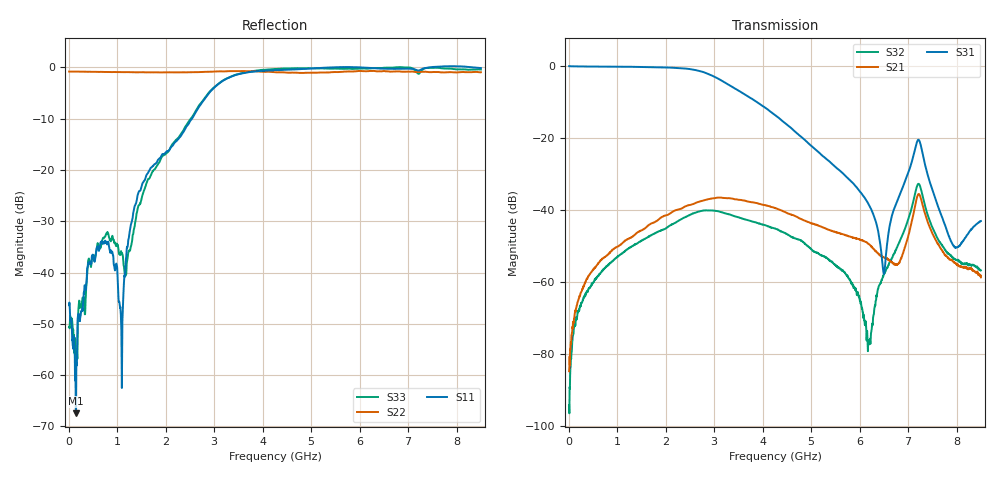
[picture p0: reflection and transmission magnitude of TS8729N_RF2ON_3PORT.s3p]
!Created with skrf (http://scikit-rf.org).
# GHz S RI R 50.0
!freq ReS11 ImS11 ReS12 ImS12 ReS13 ImS13
! ReS21 ImS21 ReS22 ImS22 ReS23 ImS23
! ReS31 ImS31 ReS32 ImS32 ReS33 ImS33
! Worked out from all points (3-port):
!   1601 points, 10 MHz to 8.5 GHz, reference 50 ohm
!   strongest paths, dB at 10 MHz, 2.132 GHz, 4.255 GHz, 6.378 GHz, 8.5 GHz:
!     S31: -0.1, -0.5, -13.6, -45.5, -43.0
!     S21: -84.7, -40.6, -39.4, -52.0, -58.6
!     S32: -94.2, -43.9, -45.1, -61.8, -56.7
!   lowest |S11| = -67.4 dB at 153.3 MHz (marker M1), VSWR 1.00, Z = 50 + j0.0217 ohm
!   |S11| at or under -10 dB: start of sweep to 2.545 GHz
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0.01  0.00455 0.00155  -1.17e-05 4.26e-05  0.9927 -0.0113
      1.37e-05 5.65e-05  -0.9094 0.00493  1.37e-05 -2.45e-05
      0.9926 -0.0114  1.9e-05 4.24e-06  0.0022 0.00197
0.1532688  -0.000365 0.000217  3.07e-05 0.000416  0.9783 -0.1229
           3.89e-05 0.000436  -0.9076 0.0485  -4.84e-05 -0.000292
           0.9783 -0.1229  -4.95e-05 -0.00031  0.000347 -0.00126
1.697388  -0.1028 -0.022  0.000863 0.00644  0.149 -0.9512
          0.000857 0.00644  -0.776 0.4434  -0.00366 0.00252
          0.1489 -0.951  -0.00367 0.00255  -0.0887 -0.006
2.742719  -0.1807 0.411  0.00942 0.00952  -0.7252 -0.4158
          0.00942 0.00949  -0.5471 0.7168  0.00281 0.00936
          -0.7254 -0.4141  0.00279 0.00935  -0.2199 0.401
4.255  0.8445 0.4066  0.00998 -0.00391  -0.1088 0.1781
       0.00998 -0.00389  -0.2796 0.8523  0.00531 -0.00151
       -0.1088 0.1775  0.00536 -0.00151  0.8125 0.5204
6.186475  0.9781 -0.1507  0.0026 -0.00221  -0.000502 0.012
          0.00258 -0.00221  0.2458 0.8849  8.26e-05 7.49e-05
          -0.000521 0.012  0.000148 3.85e-05  0.9718 -0.0846
6.494237  0.9361 -0.2554  0.00205 -0.00084  -0.00124 0.00054
          0.00206 -0.000837  0.3403 0.8539  -0.000209 0.00121
          -0.00123 0.000517  -0.000251 0.00124  0.9725 -0.1865
7.205275  0.8825 -0.2978  0.0159 0.00404  -0.0929 0.0145
          0.016 0.00403  0.5799 0.6902  0.022 0.00696
          -0.0932 0.0148  0.0219 0.00697  0.8195 -0.2863
7.937538  1.006 -0.2039  0.00157 -0.00108  -0.00266 0.00166
          0.00156 -0.00111  0.6145 0.6492  0.000677 -0.00201
          -0.00273 0.0017  0.000679 -0.00202  0.9398 -0.2083
8.5  0.9176 -0.3545  0.00112 -0.000451  -0.00541 -0.00457
     0.0011 -0.000406  0.7154 0.5383  0.000102 -0.00146
     -0.00542 -0.00452  0.000152 -0.00145  0.9063 -0.2945
